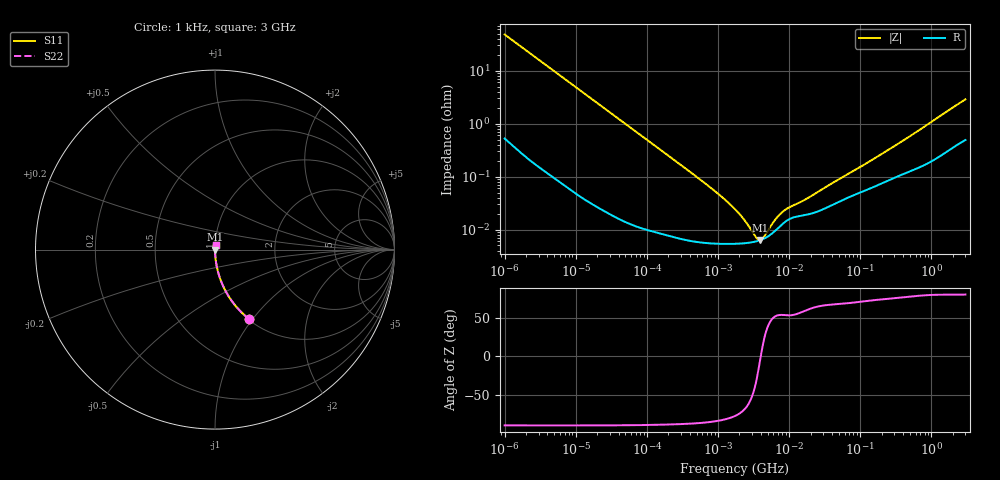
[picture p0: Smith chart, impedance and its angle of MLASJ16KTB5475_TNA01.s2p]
! MLASJ16KTB5475_TNA01  S-PARAMETER MODEL  ( Standard Model )
! Model Generated by TAIYO YUDEN Corporation (http://www.ty-top.com)
! Version 2.0
! TAIYO YUDEN Control No. 230906
! Copyright(c) 2009 TAIYO YUDEN CO.,LTD. All Rights Reserved.
! Product Description (link to TY-COMPAS)
! https://ds.yuden.co.jp/TYCOMPAS/or/detail?pn=MLASJ16KTB5475MTNA01&u=M
! Products Name : Multilayer Ceramic Capacitors
! Characteristics :
!  Capacitance : 4.7 [uF] , Rated Voltage : 6.3 [V] , TCC : X5R
!  Case Size : 1.6 x 0.8 / 0.063 x 0.031 [mm/inch] , Thickness : 0.45 / 0.018 [mm/inch]
!  (Conditions: Temperature = 25 [degC] , DC Bias Voltage = 0 [V])
! External Node Assignments :
!  1  o---| |---o  2
! GND o---------o GND
! Frequency Range : 1kHz  -  3GHz  [ 401 STEP ]
# MHZ S RI R 50
! Freq[MHz].  S11 Real  S11 Imag  S21 Real  S21 Imag  S12 Real  S12 Imag  S22 Real  S22 Imag
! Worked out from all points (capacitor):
!   401 points, 1 kHz to 3 GHz, reference 50 ohm
!   read as one part in series: C = 3.29 uF near 1.077 kHz
!   lowest |Z| = 6.32 mohm at 3.934 MHz (marker M1)
!   series resonance near 3.986 MHz, so ESL is about 490 pH
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0.001  0.1919 -0.3884  0.8081 0.3884  0.8081 0.3884  0.1919 -0.3884
0.001564  0.0899 -0.2811  0.9101 0.2811  0.9101 0.2811  0.0899 -0.2811
0.002447  0.0396 -0.1903  0.9604 0.1903  0.9604 0.1903  0.0396 -0.1903
0.004969  0.0104 -0.097  0.9896 0.097  0.9896 0.097  0.0104 -0.097
0.01216  0.00202 -0.0402  0.998 0.0402  0.998 0.0402  0.00202 -0.0402
0.033275  0.0004 -0.0148  0.9996 0.0148  0.9996 0.0148  0.0004 -0.0148
0.147855  9.65e-05 -0.00336  0.9999 0.00336  0.9999 0.00336  9.65e-05 -0.00336
0.791611  5.51e-05 -0.00061  0.9999 0.00061  0.9999 0.00061  5.51e-05 -0.00061
1.238299  5.36e-05 -0.000368  0.9999 0.000368  0.9999 0.000368  5.36e-05 -0.000368
1.732051  5.38e-05 -0.000237  0.9999 0.000237  0.9999 0.000237  5.38e-05 -0.000237
2.166294  5.46e-05 -0.000165  0.9999 0.000165  0.9999 0.000165  5.46e-05 -0.000165
2.709407  5.63e-05 -0.000101  0.9999 0.000101  0.9999 0.000101  5.63e-05 -0.000101
2.919173  5.71e-05 -8.09e-05  0.9999 8.09e-05  0.9999 8.09e-05  5.71e-05 -8.09e-05
3.14518  5.81e-05 -6.12e-05  0.9999 6.12e-05  0.9999 6.12e-05  5.81e-05 -6.12e-05
3.93371  6.31e-05 -3.35e-06  0.9999 3.35e-06  0.9999 3.35e-06  6.31e-05 -3.35e-06
4.739869  7.06e-05 4.47e-05  0.9999 -4.47e-05  0.9999 -4.47e-05  7.06e-05 4.47e-05
5.106836  7.5e-05 6.41e-05  0.9999 -6.41e-05  0.9999 -6.41e-05  7.5e-05 6.41e-05
6.881678  0.000104 0.00014  0.9999 -0.00014  0.9999 -0.00014  0.000104 0.00014
8.606987  0.000137 0.000186  0.9999 -0.000186  0.9999 -0.000186  0.000137 0.000186
21.06097  0.000202 0.000391  0.9998 -0.000391  0.9998 -0.000391  0.000202 0.000391
256.0921  0.00087 0.00317  0.9991 -0.00317  0.9991 -0.00317  0.00087 0.00317
3000  0.00567 0.028  0.9943 -0.028  0.9943 -0.028  0.00567 0.028
